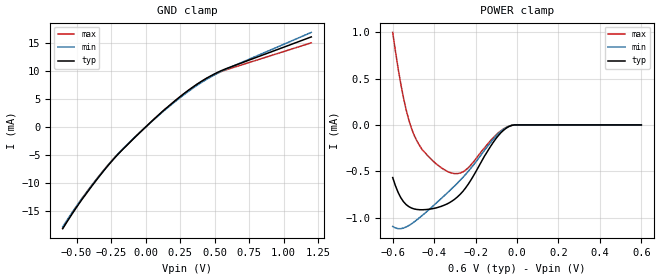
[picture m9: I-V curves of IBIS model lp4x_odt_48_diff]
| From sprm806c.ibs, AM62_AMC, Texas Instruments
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|   Model lp4x_odt_48_diff
[Model] lp4x_odt_48_diff
Model_type Input
Polarity   Non-Inverting
Enable   Active-High
Vinl =  0.0V
Vinh =  0.900V
C_comp   2.083pF   1.875pF   2.296pF
[Model Spec]
Vinh   0.900V   0.900V   0.900V
Vinl   0.0V   0.0V   0.0V
[Temperature Range]   25.000   0.125k   -40.000
[Voltage Range]   0.600V   0.570V   0.650V
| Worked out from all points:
|   GND clamp passes 1 mA (typ) near -0.04 V on its own axis
[GND_clamp]
|Voltage   I(typ)   I(min)   I(max)
-600mV    -18.2mA    -17.87mA   -18.12mA
-522mV    -15.2mA    -14.97mA   -15.03mA
-457mV    -12.85mA   -12.68mA   -12.67mA
-339mV    -8.965mA   -8.857mA   -8.835mA
-235mV    -5.847mA   -5.776mA   -5.762mA
-157mV    -3.791mA   -3.71mA    -3.752mA
26.09mV   608.8uA    579.9uA    605.7uA
143mV     3.248mA    3.129mA    3.237mA
300mV     6.401mA    6.2mA      6.381mA
430mV     8.585mA    8.377mA    8.531mA
548mV     10.1mA     9.97mA     9.941mA
1.2V      16.15mA    16.96mA    15.1mA
[POWER_clamp]
|Voltage   I(typ)   I(min)   I(max)
-600mV    -568.1uA   -1.095mA   997.9uA
-574mV    -727.9uA   -1.119mA   611.2uA
-548mV    -828uA     -1.113mA   292.2uA
-522mV    -881.9uA   -1.085mA   51.76uA
-496mV    -907uA     -1.046mA   -114.5uA
-430mV    -911.3uA   -924.2uA   -335.1uA
-326mV    -839uA     -711.5uA   -511.9uA
-287mV    -775.7uA   -626.2uA   -524.8uA
-248mV    -679.2uA   -533.6uA   -487uA
-117mV    -195.5uA   -160.4uA   -143.4uA
-39.13mV  -17.75uA   -14.14uA   -13.67uA
600mV     0A         0A         0A
